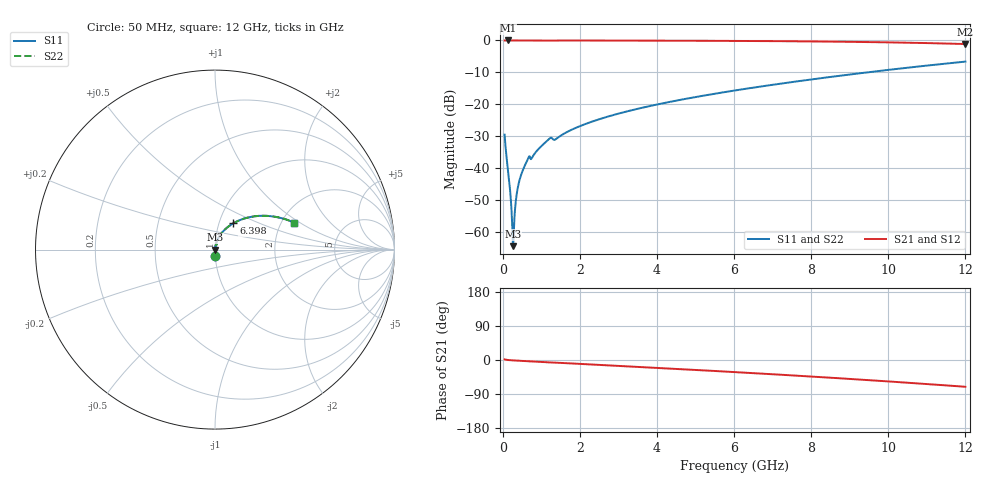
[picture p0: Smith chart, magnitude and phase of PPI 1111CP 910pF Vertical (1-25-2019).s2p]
# GHz S MA R 50
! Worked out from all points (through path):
!   1601 points, 50 MHz to 12 GHz, reference 50 ohm
!   highest |S21| = 0.00 dB at 132.2 MHz (marker M1); lowest = -1.1 dB at 12 GHz (marker M2)
!   group delay of S21, straight-line fit = 16.2 ps
!   lowest |S11| = -64.3 dB at 266.6 MHz (marker M3), VSWR 1.00, Z = 50.1 - j0.0191 ohm
!   |S11| at or under -10 dB: start of sweep to 9.44 GHz
!   |S22| runs from -64.3 to -6.6 dB; largest |S21 - S12| = 0
!   S11 on the Smith chart (normalised r, x): 50 MHz: 1.00, -0.07; 6.398 GHz: 1.17, +0.36; 12 GHz: 2.34, +0.90
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0.05  0.03374 -87.7  0.9991 1.7  0.9991 1.7  0.03374 -87.7
0.08734375  0.01792 -88.1  0.9995 0.7  0.9995 0.7  0.01792 -88.1
0.1321563  0.01008 -87.4  0.9995 0.1  0.9995 0.1  0.01008 -87.4
0.1769688  0.005672 -85.4  0.9995 -0.3  0.9995 -0.3  0.005672 -85.4
0.22925  0.002214 -76.4  0.9994 -0.7  0.9994 -0.7  0.002214 -76.4
0.2665938  0.0006098 -18.2  0.9994 -1.0  0.9994 -1.0  0.0006098 -18.2
0.289  0.001057 54.1  0.9994 -1.1  0.9994 -1.1  0.001057 54.1
0.3114062  0.001947 70.1  0.9994 -1.3  0.9994 -1.3  0.001947 70.1
0.3711563  0.004254 79.3  0.9993 -1.6  0.9993 -1.6  0.004254 79.3
0.4309062  0.006364 81.5  0.9992 -2.0  0.9992 -2.0  0.006364 81.5
0.5130625  0.009084 82.5  0.9991 -2.5  0.9991 -2.5  0.009084 82.5
0.6475  0.01374 81.5  0.9986 -3.2  0.9986 -3.2  0.01374 81.5
1.207656  0.02914 77.9  0.9965 -6.2  0.9965 -6.2  0.02914 77.9
1.371969  0.0285 76.3  0.9961 -6.8  0.9961 -6.8  0.0285 76.3
2.044156  0.04686 77.7  0.9972 -10.4  0.9972 -10.4  0.04686 77.7
2.903062  0.06923 73.6  0.9957 -14.9  0.9957 -14.9  0.06923 73.6
4.038312  0.1008 67.9  0.9926 -21.0  0.9926 -21.0  0.1008 67.9
6.025  0.1654 57.2  0.9833 -31.9  0.9833 -31.9  0.1654 57.2
6.398438  0.1792 55.1  0.9808 -34.1  0.9808 -34.1  0.1792 55.1
8.019156  0.2465 45.5  0.9655 -43.7  0.9655 -43.7  0.2465 45.5
10.01331  0.3473 32.7  0.9333 -56.6  0.9333 -56.6  0.3473 32.7
12  0.4667 18.7  0.8789 -70.7  0.8789 -70.7  0.4667 18.7
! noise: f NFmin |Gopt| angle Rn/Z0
0.05  0.0003805  0.8688  0.209  0.000624
1.372  0.006618  0.8008  5.159  0.006875
2.701  0.006642  0.6447  9.838  0.003515
4.031  0.008938  0.6158  14.44  0.004263
5.36  0.01119  0.5999  18.9  0.005023
6.682  0.01346  0.5925  23.18  0.005828
8.012  0.01584  0.5914  27.36  0.006733
9.341  0.01839  0.5958  31.4  0.007787
10.67  0.02118  0.6051  35.34  0.009053
12  0.0243  0.6186  39.2  0.01061
